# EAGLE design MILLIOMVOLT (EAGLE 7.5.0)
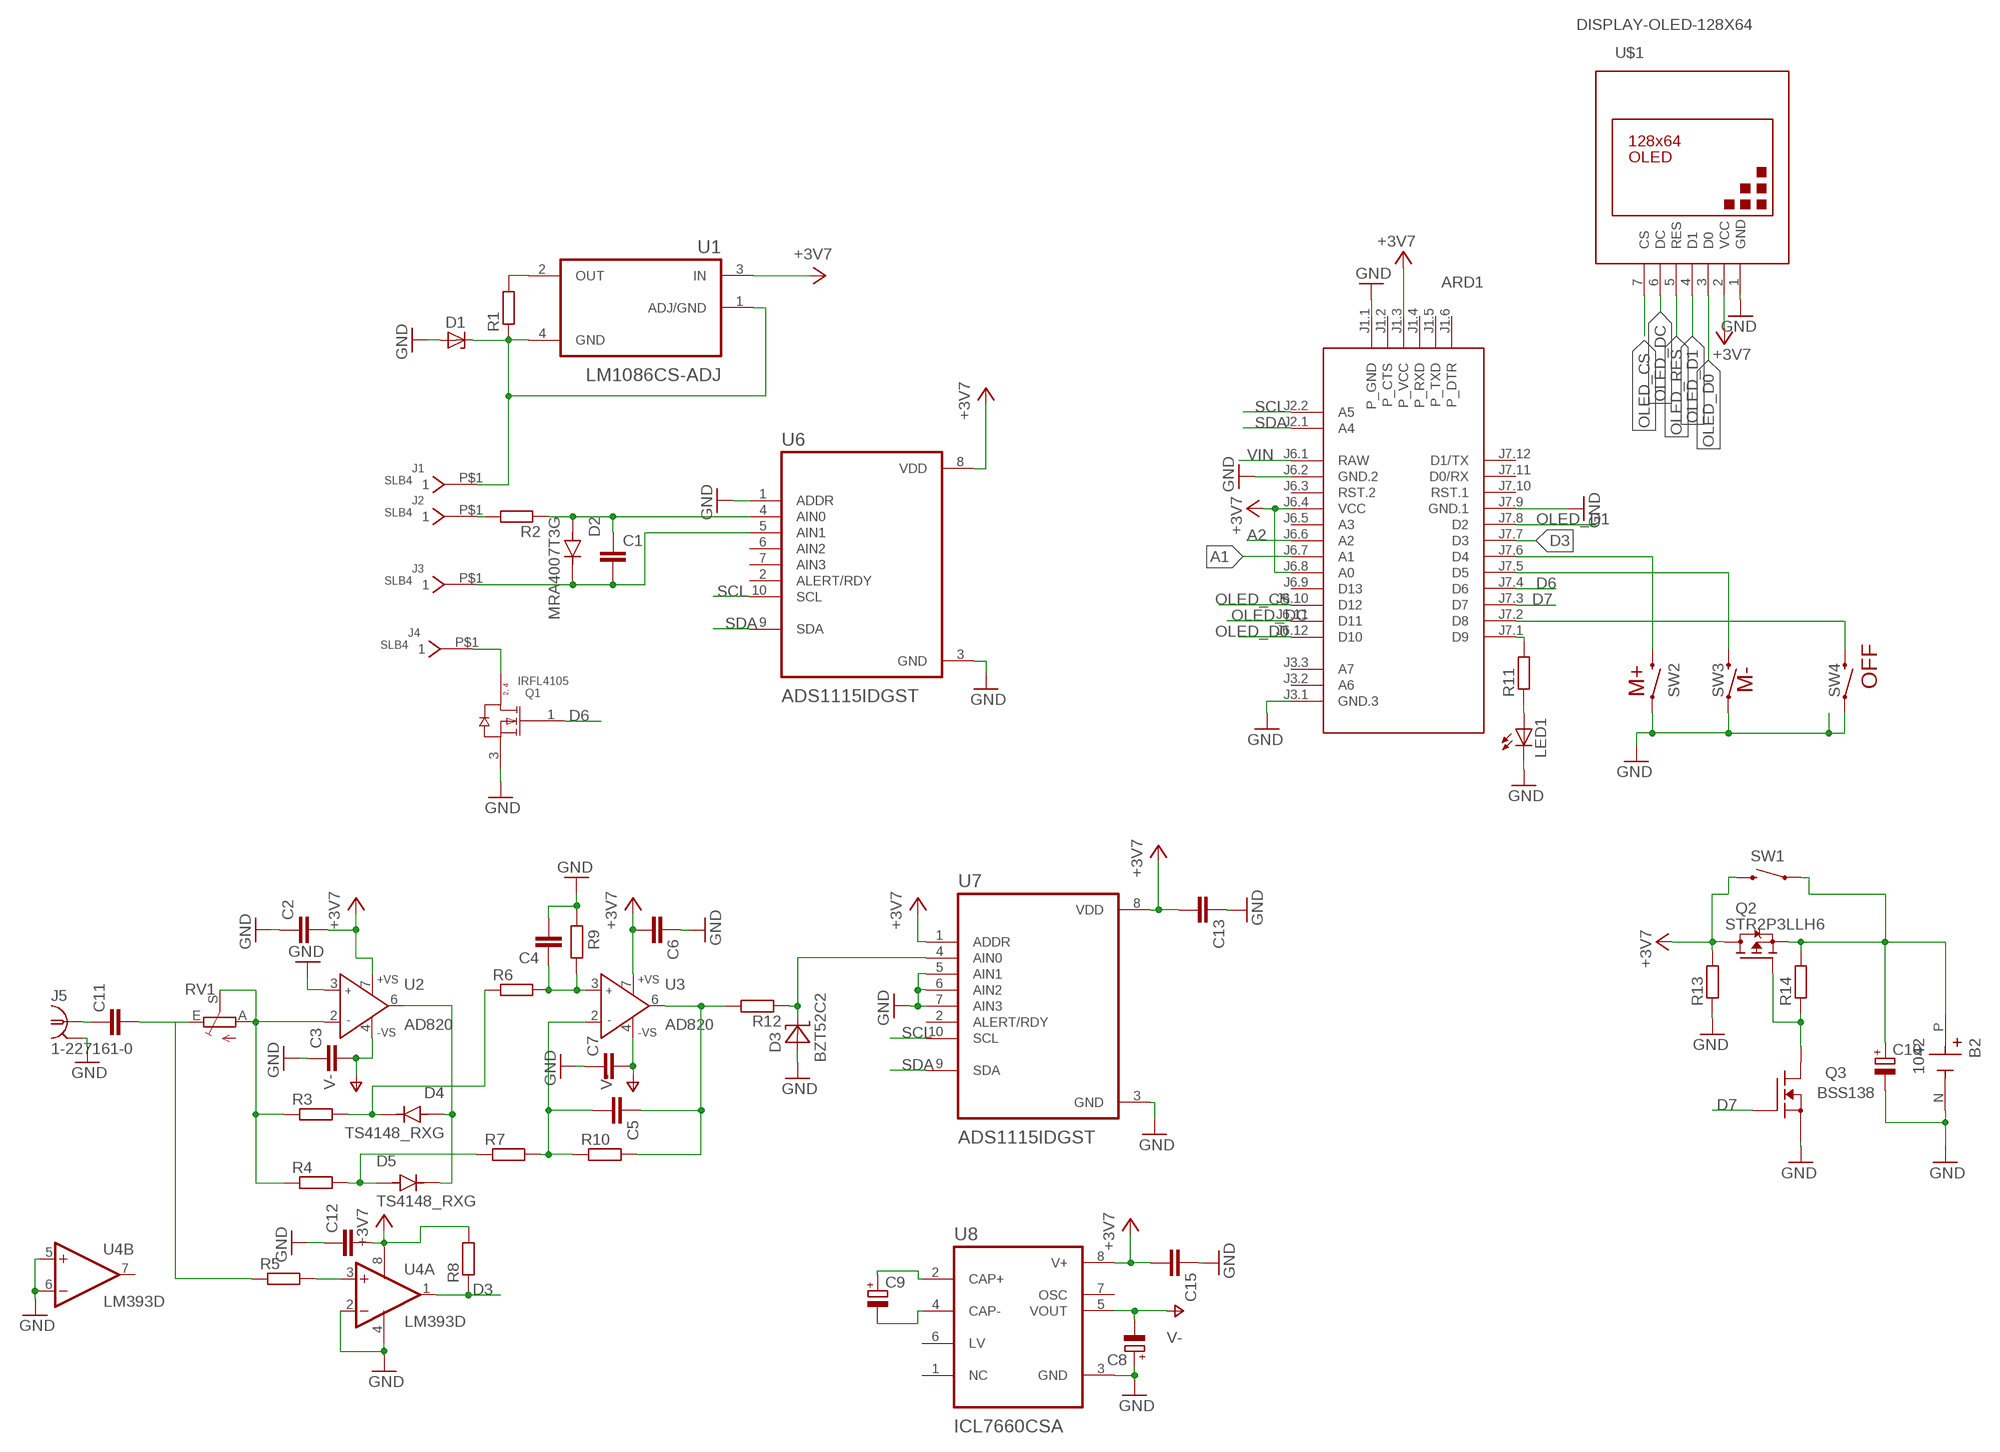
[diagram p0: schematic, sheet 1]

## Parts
ARD1  ARDUINO-PRO-MINI-3.3V  [ARDUINO-PRO-MINI]
B2  1042  [BAT_1042]
C1  C-EUC1206  [C1206]
C2  C-EUC1206  [C1206]
C3  C-EUC1206  [C1206]
C4  C-EUC1206  [C1206]
C5  C-EUC1206  [C1206]
C6  C-EUC1206  [C1206]
C7  C-EUC1206  [C1206]
C8  CPOL-EUSMCD  [SMC_D]
C9  CPOL-EUSMCD  [SMC_D]
C10  CPOL-EUSMCD  [SMC_D]
C11  C-EUC1206  [C1206]
C12  C-EUC1206  [C1206]
C13  C-EUC1206  [C1206]
C15  C-EUC1206  [C1206]
D1  ZENER-DIODESMB  [SMB]
D2  MRA4007T3G  [DIOM5226X220N]
D3  BZT52C2  [SOD123]
D4  TS4148_RXG  [DIO_TS4148_RXG]
D5  TS4148_RXG  [DIO_TS4148_RXG]
J1  SLB4  [SLB4]
J2  SLB4  [SLB4]
J3  SLB4  [SLB4]
J4  SLB4  [SLB4]
J5  1-227161-0  [AMP_227161]
LED1  LED5MM  [LED5MM]
Q1  IRFL4105  NTF3055L108T1GNTF3055L108T1G_ONSC-SOT-223-4-318E-04_V  [ONSC-SOT-223-4-318E-04_V]
Q2  STR2P3LLH6  [SOT23]
Q3  BSS138  [SOT23]
R1  R-EU_R2512  [R2512]
R2  R-EU_R2512  [R2512]
R3  R-EU_R1206  [R1206]
R4  R-EU_R1206  [R1206]
R5  R-EU_R1206  [R1206]
R6  R-EU_R1206  [R1206]
R7  R-EU_R1206  [R1206]
R8  R-EU_R1206  [R1206]
R9  R-EU_R1206  [R1206]
R10  R-EU_R1206  [R1206]
R11  R-EU_R1206  [R1206]
R12  R-EU_R1206  [R1206]
R13  R-EU_R0805  [R0805]
R14  R-EU_R0805  [R0805]
RV1  TRIM_EU-B64W  [B64W]
SW1  SWITCH-MOMENTARY-2SMD  [TACTILE-SWITCH-SMD]
SW2  SWITCH-MOMENTARY-2SMD  [TACTILE-SWITCH-SMD]
SW3  SWITCH-MOMENTARY-2SMD  [TACTILE-SWITCH-SMD]
SW4  SWITCH-MOMENTARY-2SMD  [TACTILE-SWITCH-SMD]
U1  LM1086CS-ADJ  [TO254P1524X483-4N]
U2  AD820  AD825R  [SO8]
U3  AD820  AD825R  [SO8]
U4  LM393D  [SO08]
U6  ADS1115IDGST  [SOP50P490X110-10N]
U7  ADS1115IDGST  [SOP50P490X110-10N]
U8  ICL7660CSA  [SOIC127P600X175-8N]
U$1  DISPLAY-OLED-128X64  [DISPLAY-OLED-128X64]

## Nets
+3V3: ARD1.J1.3(P_VCC) ARD1.J6.4(VCC) ARD1.J6.8(A0) C2.2 C6.2 C12.2 C13.2 C15.2 Q2.1(D) R8.2 R13.2 SW1.3 U1.3(IN) U2.7(+VS) U3.7(+VS) U4.8(P:V+) U6.8(VDD) U7.1(ADDR) U7.8(VDD) U8.8(V+) U$1.2(VCC) ; supply symbol labelled +3V7
A1: ARD1.J6.7(A1)
A2: ARD1.J6.6(A2)
D3: ARD1.J7.7(D3) R8.1 U4.1(A:OUT)
D6: ARD1.J7.4(D6) Q1.1(G)
D7: ARD1.J7.3(D7) Q3.3(G)
GND: ARD1.J1.1(P_GND) ARD1.J3.1(GND.3) ARD1.J6.2(GND.2) ARD1.J7.9(GND.1) B2.N(NEG) C2.1 C3.1 C4.2 C6.1 C7.1 C8.+ C10.- C12.1 C13.1 C15.1 D1.A D3.A J5.2 LED1.K(C) Q1.3(S) Q3.1(S) R9.2 R13.1 SW2.1 SW3.1 SW4.1 U2.3(IN+) U4.2(A:-IN) U4.4(P:V-) U4.5(B:+IN) U4.6(B:-IN) U6.1(ADDR) U6.3(GND) U7.3(GND) U7.5(AIN1) U7.6(AIN2) U7.7(AIN3) U8.3(GND) U$1.1(GND)
N$1: J2.P$1 R2.2
N$2: C1.1 D2.2(A) R2.1 U6.4(AIN0)
N$3: R1.2 U1.2(OUT)
N$4: D1.C J1.P$1 R1.1 U1.1(ADJ/GND) U1.4(GND)
N$5: C1.2 D2.1(C) J3.P$1 U6.5(AIN1)
N$6: J4.P$1 Q1.4(D)
N$7: C11.1 J5.1
N$8: C11.2 R5.1 RV1.E
N$9: R3.1 R4.1 RV1.A RV1.S U2.2(IN-)
N$10: D4.C(K) R3.2 R6.1
N$11: D5.A R4.2 R7.1
N$12: D4.A D5.C(K) U2.6(OUT)
N$13: C5.1 R10.2 R12.2 U3.6(OUT)
N$14: C4.1 R6.2 R9.1 U3.3(IN+)
N$15: C5.2 R7.2 R10.1 U3.2(IN-)
N$16: R5.2 U4.3(A:+IN)
N$17: ARD1.J7.1(D9) R11.2
N$18: ARD1.J7.6(D4) SW2.3
N$19: Q2.2(G) Q3.2(D) R14.1
N$20: B2.P(POS) C10.+ Q2.3(S) R14.2 SW1.1
N$21: LED1.A R11.1
N$22: D3.C R12.1 U7.4(AIN0)
N$23: C9.+ U8.2(CAP+)
N$24: C9.- U8.4(CAP-)
N$25: ARD1.J7.5(D5) SW3.3
N$27: ARD1.J7.2(D8) SW4.3
OLED_CS: ARD1.J6.10(D12) U$1.7(CS)
OLED_D0: ARD1.J6.12(D10) U$1.3(D0)
OLED_D1: ARD1.J7.8(D2) U$1.4(D1)
OLED_DC: ARD1.J6.11(D11) U$1.6(DC)
OLED_RES: U$1.5(RES)
SCL: ARD1.J2.2(A5) U6.10(SCL) U7.10(SCL)
SDA: ARD1.J2.1(A4) U6.9(SDA) U7.9(SDA)
V-: C3.2 C7.2 C8.- U2.4(-VS) U3.4(-VS) U8.5(VOUT)
VIN: ARD1.J6.1(RAW)
Unconnected: ARD1.J1.2(P_CTS) ARD1.J1.4(P_RXD) ARD1.J1.5(P_TXD) ARD1.J1.6(P_DTR) ARD1.J3.2(A6) ARD1.J3.3(A7) ARD1.J6.3(RST.2) ARD1.J6.5(A3) ARD1.J6.9(D13) ARD1.J7.10(RST.1) ARD1.J7.11(D0/RX) ARD1.J7.12(D1/TX) Q1.2(D) U4.7(B:OUT) U6.2(ALERT/RDY) U6.6(AIN2) U6.7(AIN3) U7.2(ALERT/RDY) U8.1(NC) U8.6(LV) U8.7(OSC)

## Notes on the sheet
- M- | OFF
- M+

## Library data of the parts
ARD1 = diy-modules:ARDUINO-PRO-MINI-*: Arduino Pro Mini and compatible devices More details available here: https://www.arduino.cc/en/Main/ArduinoBoardProMini Click here to find device on ebay.com
B2 = 18650-HOLDER:1042: Check availability; AVAILABILITY: In Stock; CHECK_PRICES: https://www.snapeda.com/parts/1042/Keystone/view-part/?ref=eda; DESCRIPTION: SMT Holder for 18650 Battery; MF: Keystone Electronics Corp.; MP: 1042; PACKAGE: NON STANDARD-5 Keystone; PRICE: None; SNAPEDA_LINK: https://www.snapeda.com/parts/1042/Keystone/view-part/?ref=snap
C1-C7 C11-C13 C15 = rcl:C-EU: CAPACITOR, European symbol
C8-C10 = rcl:CPOL-EU: POLARIZED CAPACITOR, European symbol
D1 = diode:ZENER-DIODE: Z-Diode
D2 = MRA4007T3G:MRA4007T3G: Check availability; AVAILABILITY: In Stock; CHECK_PRICES: https://www.snapeda.com/parts/MRA4007T3G/Onsemi/view-part/?ref=eda; DESCRIPTION: Diode Standard 1000 V 1A Surface Mount SMA; MF: ON Semiconductor; MP: MRA4007T3G; PACKAGE: SMA-2 ON Semiconductor; PRICE: None; SNAPEDA_LINK: https://www.snapeda.com/parts/MRA4007T3G/Onsemi/view-part/?ref=snap
D3 = diode:BZT52C2
D4 D5 = TS4148_RXG:TS4148_RXG: Check availability Check availability Check availability; AVAILABILITY: In Stock; CHECK_PRICES: https://www.snapeda.com/parts/TS4148%20RXG/Taiwan+Semiconductor/view-part/?ref=eda; DESCRIPTION: 1206 (Ceramics) 75V 0.15A Switching Diode & Array; MF: Taiwan Semiconductor; MP: TS4148 RXG; PACKAGE: 1206-2 Taiwan Semiconductor; PRICE: None; SNAPEDA_LINK: https://www.snapeda.com/parts/TS4148%20RXG/Taiwan+Semiconductor/view-part/?ref=snap
J1-J4 = con-jack:SLB4: Bananas socket PCB
J5 = con-coax:?227161*: JACK, RIGHT ANGLE, 50 OHM, PCB, BNC; MF: TYCO ELECTRONICS; MPN: 1-227161; OC_FARNELL: unknown; OC_NEWARK: 33B3200
LED1 = led:LED: LED
Q1 = NTF3055L108T1G:NTF3055L108T1G: Power MOSFET, 3 A, 60 V, Logic Level, N-Channel, 4-Pin SOT-223, Pb-Free, Tape and Reel Check availability; AVAILABILITY: In Stock; CHECK_PRICES: https://www.snapeda.com/parts/NTF3055L108T1G/Onsemi/view-part/?ref=eda; DESCRIPTION: N-Channel 60 V 3A (Ta) 1.3W (Ta) Surface Mount SOT-223 (TO-261); MF: ON Semiconductor; MP: NTF3055L108T1G; PACKAGE: SOT-223-4 ON Semiconductor; PRICE: None; SNAPEDA_LINK: https://www.snapeda.com/parts/NTF3055L108T1G/Onsemi/view-part/?ref=snap
Q2 = transistor-fet:STR2P3LLH6
Q3 = transistor-fet:BSS138
R1-R14 = rcl:R-EU_: RESISTOR, European symbol
RV1 = pot:TRIM_EU-: POTENTIOMETER
SW1-SW4 = SparkFun-Electromechanical:SWITCH-MOMENTARY-2: Various NO switches- pushbuttons, reed, etc; PROD_ID: SWCH-08247
U1 = LM1086CS-ADJ:LM1086CS-ADJ: Check availability; AVAILABILITY: In Stock; CHECK_PRICES: https://www.snapeda.com/parts/LM1086CS-ADJ/NOPB/Texas+Instruments/view-part/?ref=eda; DESCRIPTION: 1.5-A, 29-V, linear voltage regulator; MF: Texas Instruments; MP: LM1086CS-ADJ/NOPB; PACKAGE: TO263-3 Texas Instruments; PRICE: None; SNAPEDA_LINK: https://www.snapeda.com/parts/LM1086CS-ADJ/NOPB/Texas+Instruments/view-part/?ref=snap
U2 U3 = analog-devices:AD825: Low Cost, General-Purpose High Speed JFET Amplifier Source: http://www.analog.com/static/imported-files/data_sheets/AD825.pdf; MF: ALTERA CORPORATION; MPN: AD825ARZ; OC_FARNELL: 9603735; OC_NEWARK: 59K6528
U4 = linear:LM393: COMPARATOR
U6 U7 = ADS1115IDGST:ADS1115IDGST: Check availability; AVAILABILITY: In Stock; CHECK_PRICES: https://www.snapeda.com/parts/ADS1115IDGST/Texas+Instruments/view-part/?ref=eda; DESCRIPTION: 16-bit, 860-SPS, 4-channel, delta-sigma ADC with PGA, oscillator, VREF, comparator and I2C; MF: Texas Instruments; MP: ADS1115IDGST; PACKAGE: VSSOP-10 Texas Instruments; PRICE: None; SNAPEDA_LINK: https://www.snapeda.com/parts/ADS1115IDGST/Texas+Instruments/view-part/?ref=snap
U8 = ICL7660CSA:ICL7660CSA: Check availability; AVAILABILITY: In Stock; CHECK_PRICES: https://www.snapeda.com/parts/ICL7660CSA/Analog+Devices/view-part/?ref=eda; DESCRIPTION: Charge Pump Switching Regulator IC Positive or Negative Fixed -Vin, nVin, Vin/2 1 Output 20mA 8-SOIC (0.154, 3.90mm Width); MF: Analog Devices; MP: ICL7660CSA; PACKAGE: SOIC-8 Maxim; PRICE: None; SNAPEDA_LINK: https://www.snapeda.com/parts/ICL7660CSA/Analog+Devices/view-part/?ref=snap
U$1 = diy-modules:DISPLAY-OLED-128X64: 128x64 Dot Matrix OLED Module based on SSD1306 chip Variant with SPI interface More details available here: http://www.instructables.com/id/How-to-use-OLED-display-arduino-module/ SSD1306 datasheet: https://cdn-shop.adafruit.com/datasheets/SSD1306.pdf Click here to find device on ebay.com Note: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

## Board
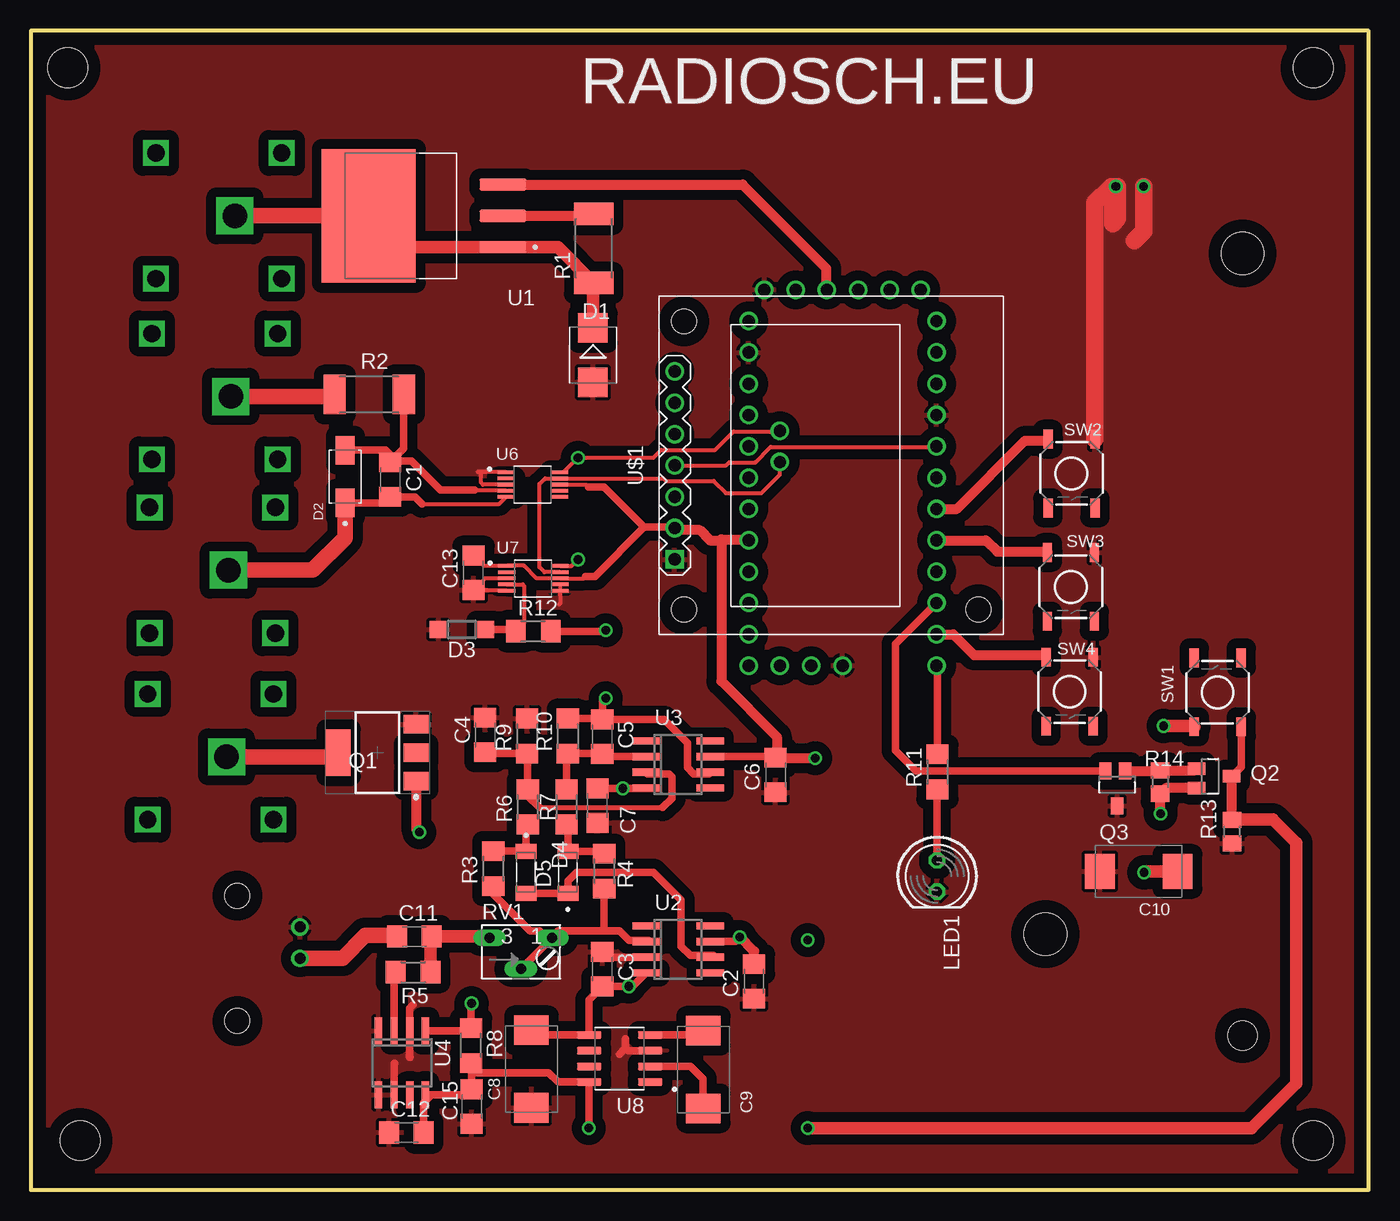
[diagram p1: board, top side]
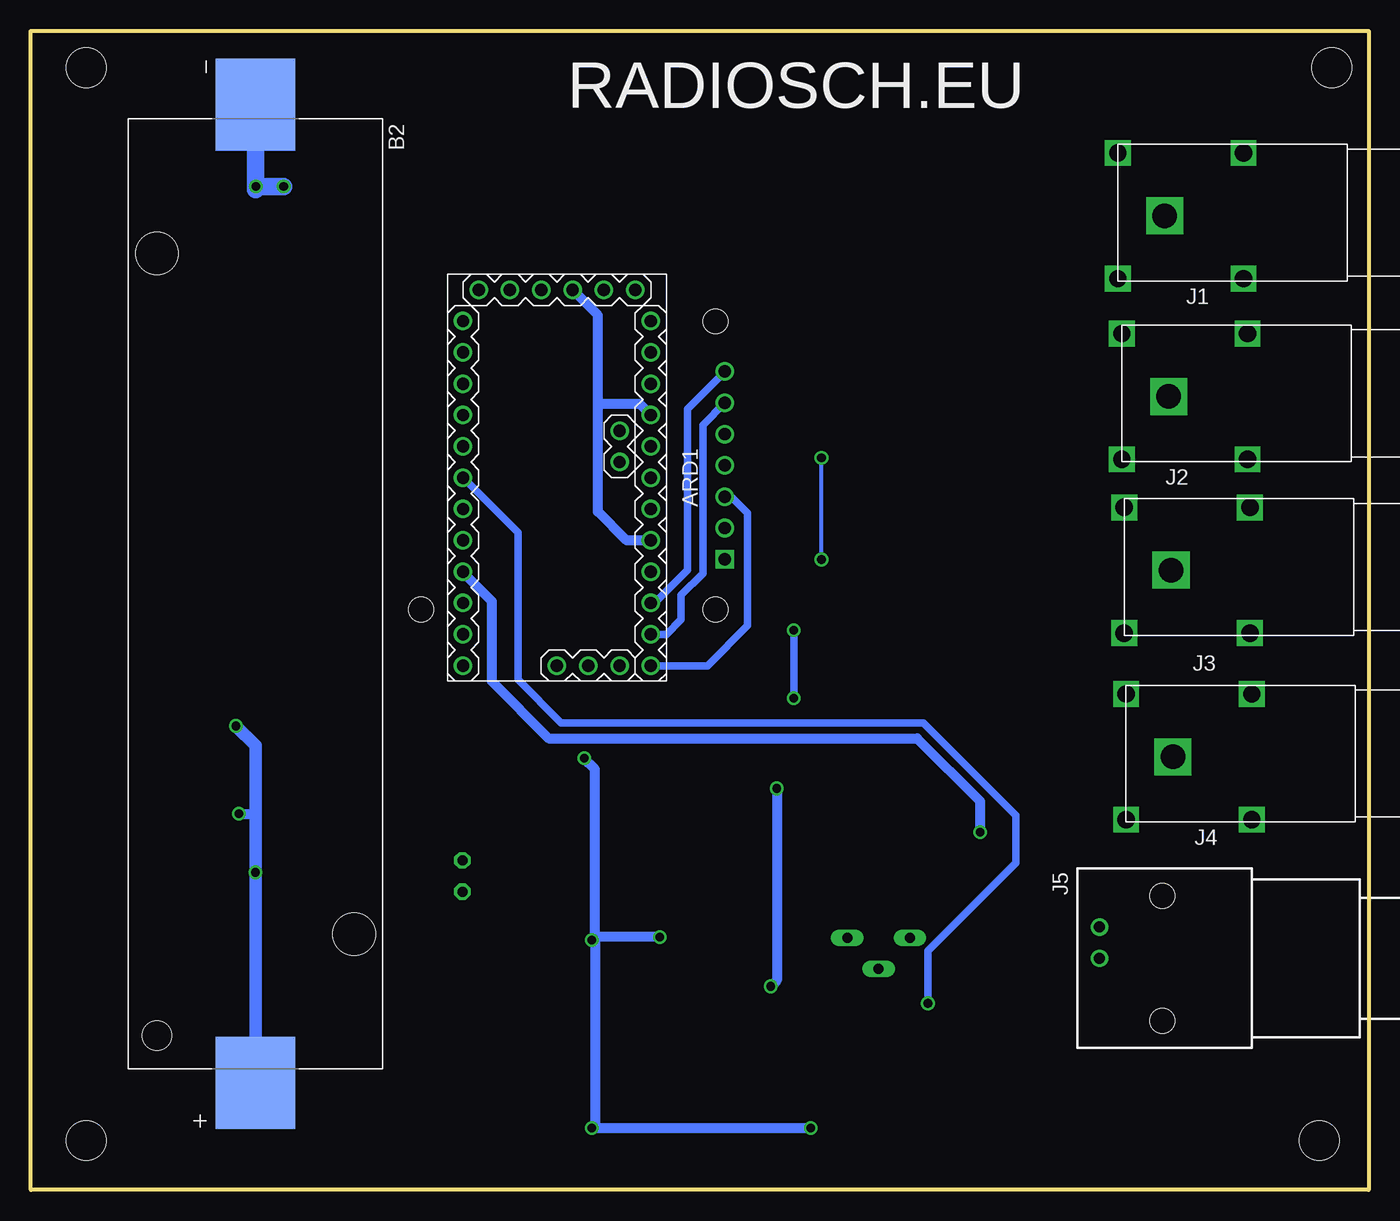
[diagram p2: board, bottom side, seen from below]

Size 108.5 x 94 mm. Coordinates in mm from the lower left corner, seen from the top.
Outline: 0,0 108.5,0 108.5,94 0,94 0,0
Copper layers (1*16): Top 0.035mm / dielectric 1.5mm / Bottom 0.035mm
Design rules "default *": minimum track width 10mil, minimum drill 24mil, track to track 6mil, track to pad 6mil, pad to pad 6mil, via to via 8mil, smd to smd 8mil, copper to edge 40mil, drill to drill 8mil, minimum pad ring 10mil, minimum via ring 8mil, stop-mask expansion 4mil, vias tented up to drill 0mil, thermal gap 10mil
Holes 3.2 mm at 3,91 4,4 104,4 104,91

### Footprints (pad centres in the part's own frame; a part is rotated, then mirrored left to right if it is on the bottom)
ARDUINO-PRO-MINI = drill 1: J1.1 -15.24,6.35; J1.2 -15.24,3.81; J1.3 -15.24,1.27; J1.4 -15.24,-1.27; J1.5 -15.24,-3.81; J1.6 -15.24,-6.35; J2.1 -1.27,5.08; J2.2 -3.81,5.08; J3.1 15.24,0; J3.2 15.24,2.54; J3.3 15.24,5.08; J6.1 -12.7,7.62; J6.2 -10.16,7.62; J6.3 -7.62,7.62; J6.4 -5.08,7.62; J6.5 -2.54,7.62; J6.6 0,7.62; J6.7 2.54,7.62; J6.8 5.08,7.62; J6.9 7.62,7.62; J6.10 10.16,7.62; J6.11 12.7,7.62; J6.12 15.24,7.62; J7.1 15.24,-7.62; J7.2 12.7,-7.62; J7.3 10.16,-7.62; J7.4 7.62,-7.62; J7.5 5.08,-7.62; J7.6 2.54,-7.62; J7.7 0,-7.62; J7.8 -2.54,-7.62; J7.9 -5.08,-7.62; J7.10 -7.62,-7.62; J7.11 -10.16,-7.62; J7.12 -12.7,-7.62
BAT_1042 = smd 7.46 x 6.47: N -39.67,0; P 39.67,0 | hole 3.45: 27.6,8; -27.6,-8 | hole 2.39: 35.82,-8
C1206 = smd 1.6 x 1.8: 1 -1.4,0; 2 1.4,0
SMC_D = smd 2.4 x 2.8: + -3.15,0; - 3.15,0
SMB = smd 2.4 x 2.4: A 2.2,0; C -2.2,0
DIOM5226X220N = smd 2.31 x 1.54: 1 -2.145,0; 2 2.145,0
SOD123 = smd 1.4 x 1.4: A 1.9,0; C -1.9,0
DIO_TS4148_RXG = smd 1.2 x 1.7: A 1.7,0; C -1.7,0
SLB4 = drill 2 square: P$1 0,0 | drill 1.4 square: P$2 3.8,-5.1; P$3 3.8,5.1; P$4 -6.4,5.1; P$5 -6.4,-5.1
AMP_227161 = drill 0.9 pad 1.27: 1 0,-5.08; 2 -2.54,-5.08 | hole 2: -5.08,0; 5.08,0
LED5MM = drill 0.813 octagon: A -1.27,0; K 1.27,0
ONSC-SOT-223-4-318E-04_V = smd 2 x 1.5: 1 -3.15,2.3; 2 -3.15,0; 3 -3.15,-2.3 | smd 2 x 3.8: 4 3.15,0
SOT23 = smd 1 x 1.4: 1 0,1.735; 2 -0.632,-1.1; 3 0.95,-1.1
R2512 = smd 1.8 x 3.2: 1 -2.8,0; 2 2.8,0
R1206 = smd 1.6 x 1.803: 1 -1.422,0; 2 1.422,0
R0805 = smd 1.3 x 1.5: 1 -0.95,0; 2 0.95,0
B64W = drill 0.813 long: A 2.54,0; E -2.54,0; S 0,-2.54
TACTILE-SWITCH-SMD = smd 1.524 x 0.762: 1 -2.794,1.905; 2 2.794,1.905; 3 -2.794,-1.905; 4 2.794,-1.905
TO254P1524X483-4N = smd 3.79 x 0.99: 1 -6.4,2.54; 2 -6.4,0; 3 -6.4,-2.54 | smd 7.62 x 10.84: 4 4.48,0
SO8 = smd 0.6 x 2.2: 1 -1.905,-2.6; 2 -0.635,-2.6; 3 0.635,-2.6; 4 1.905,-2.6; 5 1.905,2.6; 6 0.635,2.6; 7 -0.635,2.6; 8 -1.905,2.6
SO08 = smd 0.6 x 2.2: 1 -1.905,-2.6; 2 -0.635,-2.6; 3 0.635,-2.6; 4 1.905,-2.6; 5 1.905,2.6; 6 0.635,2.6; 7 -0.635,2.6; 8 -1.905,2.6
SOP50P490X110-10N = smd 1.47 x 0.28: 1 -2.15,1; 2 -2.15,0.5; 3 -2.15,0; 4 -2.15,-0.5; 5 -2.15,-1; 6 2.15,-1; 7 2.15,-0.5; 8 2.15,0; 9 2.15,0.5; 10 2.15,1
SOIC127P600X175-8N = smd 1.97 x 0.59: 1 -2.475,1.905; 2 -2.475,0.635; 3 -2.475,-0.635; 4 -2.475,-1.905; 5 2.475,-1.905; 6 2.475,-0.635; 7 2.475,0.635; 8 2.475,1.905
DISPLAY-OLED-128X64 = drill 1 square: 1 -7.62,12.7 | drill 1: 2 -5.08,12.7; 3 -2.54,12.7; 4 0,12.7; 5 2.54,12.7; 6 5.08,12.7; 7 7.62,12.7 | hole 2: -11.684,11.938; 11.684,11.938; -11.684,-11.938

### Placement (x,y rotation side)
ARD1  65.83,57.76 270 bottom
B2  90.28,48.34 270 bottom
C1  29.15,57.6 270 top
C2  58.65,16.9 90 top
C3  46.35,17.9 270 top
C4  36.85,36.9 90 top
C5  46.35,36.75 270 top
C6  60.4,33.65 90 top
C7  45.95,31.15 90 top
C8  40.6,9.8 90 top
C9  54.55,9.75 90 top
C10  89.85,25.82 180 top
C11  31.1,20.55 0 top
C12  30.45,4.65 0 top
C13  35.9,50.05 90 top
C15  35.75,6.75 90 top
D1  45.59,67.69 270 top
D2  25.5,57.85 90 top
D3  34.95,45.45 180 top
D4  40.15,25.75 270 top
D5  43.55,25.75 90 top
J1  16.55,79 180 bottom
J2  16.23,64.35 180 bottom
J3  16.02,50.25 180 bottom
J4  15.88,35.12 180 bottom
J5  16.75,18.77 270 bottom
LED1  73.5,25.45 270 top
Q1  28.1,35.45 180 top
Q2  95.64,33.53 270 top
Q3  88.1,32.87 180 top
R1  45.65,76.35 90 top
R2  27.45,64.5 180 top
R3  37.5,26.05 90 top
R4  46.5,25.85 90 top
R5  31,17.65 180 top
R6  40.3,31.05 90 top
R7  43.45,31.05 90 top
R8  35.7,11.7 270 top
R9  40.25,36.8 90 top
R10  43.55,36.8 90 top
R11  73.53,33.9 90 top
R12  40.75,45.3 0 top
R13  97.42,29.05 90 top
R14  91.58,33.08 270 top
RV1  39.75,20.45 0 top
SW1  96.25,40.35 90 top
SW2  84.4,58.1 270 top
SW3  84.35,48.9 270 top
SW4  84.25,40.4 270 top
U1  31.88,78.99 180 top
U2  52.5,19.5 270 top
U3  52.5,34.5 270 top
U4  30.1,10.3 180 top
U6  40.7,57.2 0 top
U7  40.75,49.6 0 top
U8  47.75,10.65 180 top
U$1  64.91,58.75 90 top

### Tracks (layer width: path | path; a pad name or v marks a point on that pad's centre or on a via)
+3V3  (via drill 0.7)
  Top 0.305: U6.8 45.05,57.2 45.25,57 | 45,49.75 44.85,49.6 U7.8 41.02,49.6 40,50.62 38.62,50.62 U7.1 36.75,50.6 C13.2
  Top 0.61: U4.8 32.5,7.7 | 32.5,7.7 35.3,7.7 C15.2 35.75,9.5 | C12.2 31.85,7.05 32.5,7.7 | 35.75,9.5 35.75,10.23 R8.2 | U8.8 42.76,8.74 42,9.5 35.75,9.5 | U8.8 45.27,5.73 | 60.38,35.03 C6.2 60.31,35.14 U3.7 | U8.8 45.27,5.02 v45.25,5 | U2.7 57.13,20.13 v57.5,20.5 | 45.25,57 46.5,57 49.75,53.75 | 49.75,53.75 52.13,53.75 U$1.2 | 45,49.75 45.75,49.75 49.75,53.75 | SW1.3 98.16,34.31 Q2.1 | 97.38,30.04 R13.2
  Top 0.813: 57.34,20.34 v57.5,20.5 58.65,19.35 C2.2 | U$1.2 52.38,53.5 54.25,53.5 55.07,52.68 55.93,52.68 56,52.75 | 56,52.75 56,41.25 60.5,36.75 60.5,35.15 C6.2 60.45,35 v63.62,35 | 56,52.75 58.14,52.75 ARD1.J6.8 | U1.3 57.72,81.53 64.5,74.75 64.5,73.06 ARD1.J1.3 | 97.38,30.04 Q2.1
  Top 1.016: 97.38,30.04 100.71,30.04 102.62,28.12 102.62,8.62 99,5 v63,5
  Bottom 0.813: v45.25,5 v63,5 62.75,5.25 62.75,20.5 | v57.5,20.5 62.75,20.5 | 62.75,20.5 v63,20.25 | ARD1.J6.8 60.18,52.68 62.5,55 62.5,64 | 62.5,64 62.5,70.94 ARD1.J1.3 | ARD1.J6.4 59.12,63.75 62.25,63.75 62.5,64 | 62.75,20.5 62.75,34.12 v63.62,35
D3  (via drill 0.7)
  Top 0.61: U4.1 35.48,12.9 R8.1 35.7,15.08 v35.75,15.12
  Bottom 0.61: v35.75,15.12 35.75,19.38 28.62,26.5 28.62,30.38 36.12,37.88 65.5,37.88 69,41.38 69,53.31 ARD1.J7.7
D6  (via drill 0.7)
  Top 0.813: Q1.1 31.25,29.25 v31.5,29
  Bottom 0.813: v31.5,29 31.5,31.5 36.62,36.62 66.5,36.62 71.12,41.25 71.12,47.75 73.45,50.08 ARD1.J7.4
D7
  Top 0.61: Q3.3 71.78,33.97 70.12,35.62 70.12,44.27 ARD1.J7.3
GND  (via drill 0.7)
  Top 0.305: U7.7 U7.6 42.9,47.52 42.88,47.5 | U6.1 36.62,58.2 | 36.62,58.2 36.3,58.2 36.25,58.25 | U6.3 36.67,57.2 36.5,57.38 36.5,58.08 36.62,58.2 | U7.3 36.85,49.6 C13.1 35.95,48.6 U7.5
  Top 0.61: 31,15 30.73,14.73 U4.2 30.73,10.77 30.75,10.75 | 46.59,19.06 C3.1 46.78,18.87 U2.3 | U8.3 48.47,11.28 48.25,11.5 | 48.25,11.5 47.75,11 | U4.6 29.46,10.22 29.5,10.25 | 48.25,11.5 48.25,12.25
  Top 1.422: v90.25,81.38 90.25,77.75 89.5,77 | SW2.1 86.31,80.06 87.62,81.38 v88,81.38 | v88,81.38 88.12,81.38 88.12,78.75 87.75,78.38 87.75,81.12 v88,81.38
  Bottom 1.422: B2.N 90.28,81.28 v90.25,81.38 | v88,81.38 90,81.38 90.25,81.12
  pour Top (isolate 0.813): 1,93.5 107.5,93.5 107.5,1.5 1,1.5
N$1
  Top 0.813: 24.55,64.4 R2.2
  Top 1.27: J2.P$1 24.5,64.35 R2.2
N$2
  Top 0.305: U6.4 36.05,56.7 36,56.75
  Top 0.61: 36,56.75 33.25,56.75 30.88,59.12 29.62,59.12 | 29.62,59.12 28.75,59.12 28.62,59.25 28.9,59.25 C1.1 30.25,60.1 R2.1 | D2.2 28.75,59.99 29.62,59.12
N$3
  Top 0.813: U1.2 45.49,78.99 R1.2
N$4
  Top 1.016: U1.4 29.94,76.45 U1.1 42.75,76.45 R1.1 45.59,73.49 D1.C
  Top 1.27: J1.P$1 U1.4
N$5
  Top 0.305: 31.75,55.62 37.98,55.62 U6.5
  Top 0.61: C1.2 29.75,56.2 | 29.75,56.2 31.18,56.2 31.75,55.62 | D2.1 29.25,55.7 29.75,56.2
  Top 1.27: J3.P$1 22.88,50.25 25.5,52.88 D2.1
N$6
  Top 1.016: 24.75,35.25 Q1.4
  Top 1.27: J4.P$1 24.62,35.12 Q1.4
N$7
  Top 1.016: 29.65,20.5 C11.1
  Top 1.27: J5.1 25.27,18.77 27.12,20.62 29.62,20.62 C11.1
N$8
  Top 1.016: RV1.E 37.11,20.55 C11.2 32.42,20.47 R5.1
N$9
  Top 0.406: 50.1,20.25 49.9,20.25 U2.2
  Top 0.61: RV1.A 42.29,20.54 42.75,21 46.25,21 | 46.25,21 47.75,21 48.5,20.25 50.1,20.25 | R3.1 37.5,24 40.5,21 41.25,21 41.75,20.5 42.24,20.5 RV1.A | RV1.S RV1.A | R4.1 46.5,21.25 46.25,21
N$10
  Top 0.61: R3.2 40.13,27.47 D4.C 40.15,29.48 R6.1
N$11
  Top 0.61: R4.2 46.32,27.45 D5.A 43.55,29.53 R7.1
N$12
  Top 0.406: U2.6 55,18.87 55,19
  Top 0.61: D4.A D5.C 43.55,25.05 44.25,25.75 50.5,25.75 52.75,23.5 52.75,19.75 53.5,19 55,19 55.35,19
N$13  (via drill 0.7)
  Top 0.61: R10.2 46.28,38.22 C5.1 | C5.1 51.35,38.15 53.25,36.25 53.25,34.25 53.75,33.75 54.98,33.75 U3.6 | R12.2 46.55,45.3 v46.62,45.38 | C5.1 46.35,39.6 v46.62,39.88
  Bottom 0.61: v46.62,39.88 v46.62,45.38
N$14
  Top 0.406: 41.25,31 51.25,31
  Top 0.61: C4.1 36.97,35.38 R9.1 40.3,35.33 R6.2 40.3,31.95 41.25,31 | 51.25,31 52,31.75 52,33.5 51.75,33.75 50.02,33.75 U3.3
N$15
  Top 0.61: R7.2 43.45,35.28 R10.1 46.32,35.38 C5.2 46.56,35.14 U3.2
N$16
  Top 0.61: U4.3 29.46,17.54 R5.2
N$17
  Top 0.61: R11.2 73.53,42.45 ARD1.J7.1
N$18
  Top 0.813: ARD1.J7.6 75.09,55.22 80.62,60.75 82.35,60.75 SW2.3
N$19
  Top 0.813: Q3.2 91.52,33.97 R14.1 94.41,34.03 Q2.2
N$20  (via drill 0.7)
  Top 0.813: Q2.3 92.03,32.59 R14.2 91.58,30.55 v91.62,30.5
  Top 1.016: v91.88,37.62 94.28,37.62 SW1.1 | C10.+ 90.36,25.82 v90.28,25.75
  Bottom 0.813: v91.62,30.5 90.41,30.5 90.28,30.38
  Bottom 1.016: B2.P v90.28,25.75 90.28,30.38 90.28,36.03 v91.88,37.62
N$21
  Top 0.61: LED1.A 73.5,32.45 R11.1
N$22
  Top 0.305: U7.4 39.9,49.1 40,49 40,45.97 R12.1
  Top 0.61: D3.C 39.18,45.45 R12.1
N$23
  Top 0.61: U8.2 53.48,10.02 54.5,9 54.5,6.65 C9.+
N$24
  Top 0.61: U8.4 54.2,12.55 C9.-
N$25
  Top 0.813: ARD1.J7.5 77.44,52.68 78.38,51.75 82.39,51.75 SW3.3
N$27
  Top 0.813: ARD1.J7.2 74.81,45.06 76.5,43.38 82.16,43.38 SW4.3
OLED_CS
  Bottom 0.61: ARD1.J6.10 57.9,47.6 55.25,50.25 55.25,63.33 U$1.7
OLED_D0
  Bottom 0.61: U$1.3 51.71,56.21 50.38,54.88 50.38,45.75 53.62,42.5 58.19,42.5 ARD1.J6.12
OLED_D1
  Top 0.305: U$1.4 56.38,58.75 56.62,59 58.75,59 60,60.25 73.4,60.25 ARD1.J7.8
OLED_DC
  Bottom 0.61: ARD1.J6.11 56.94,45.06 55.75,46.25 55.75,48.25 54,50 54,62.04 U$1.6
SCL  (via drill 0.7)
  Top 0.305: U7.10 43.85,50.6 v44.38,51.12 | ARD1.J2.2 60.68,61.5 57,61.5 55.5,60 51.12,60 50.5,59.38 v44.38,59.38 43.2,58.2 U6.10
  Bottom 0.305: v44.38,51.12 v44.38,59.38
SDA
  Top 0.305: U7.9 41.65,50.1 41.25,50.5 41.25,57.25 41.62,57.62 41.66,57.62 41.73,57.69 42.84,57.69 U6.9 51.3,57.7 51.5,57.5 55.38,57.5 56.38,56.5 59.25,56.5 60.75,58 ARD1.J2.1
V-  (via drill 0.7)
  Top 0.61: C8.- 40.99,12.55 U8.5 45.27,15.42 C3.2 v48.5,16.5 48.8,16.5 U2.4 | 49.95,32.55 v48,32.55 C7.2 | 50.88,32.55 49.95,32.55 | 49.95,32.55 U3.4
  Bottom 0.813: v48,32.55 48,17 v48.5,16.5

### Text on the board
tPlace: RADIOSCH.EU
bPlace: RADIOSCH.EU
